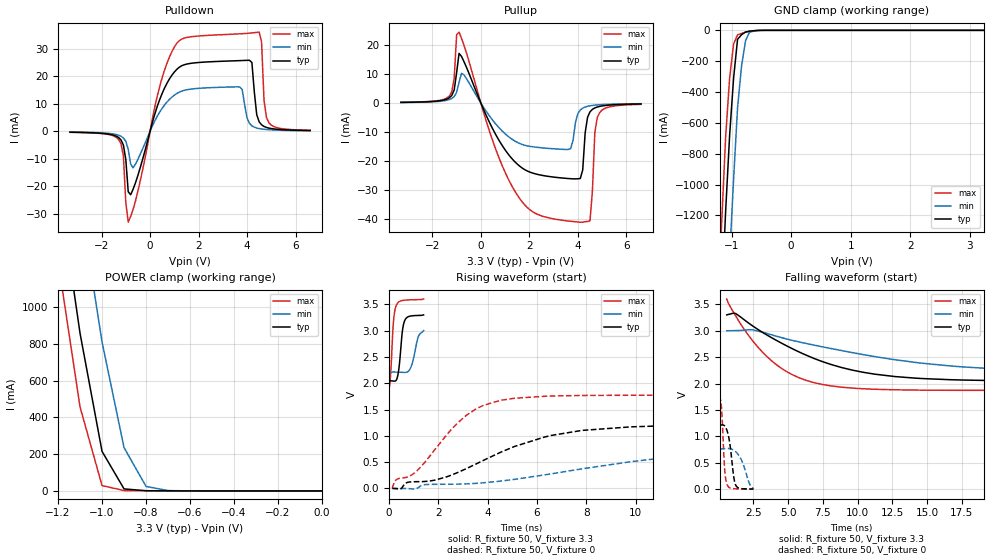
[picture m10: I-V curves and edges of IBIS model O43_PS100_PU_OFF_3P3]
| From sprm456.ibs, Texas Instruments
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|   Model Cell O43_PS100_PU_OFF_3P3
|IDG09_OUO43_PS100_PU_OFF_3P3
[Model]   O43_PS100_PU_OFF_3P3
Model_type   I/O
Polarity   Non-Inverting
Enable   Active-Low
Vinl =  0.8V
Vinh =  2V
Cref =  15pF
Rref =  100.00M
Vref =  0V
Vmeas =  1.65
C_comp   1.7423p   1.5272001p   2.1795998p
[Model Spec]
Vinl   0.8V   0.8V   0.8V
Vinh   2V   2V   2V
[Temperature Range]   25   125   -40
[Voltage Range]   3.3   3   3.6
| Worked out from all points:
|   slope of the pulldown table from 0 to 0.495 V, typ, clamps not added: 36.1 ohm
|   slope of the pullup table from 0 to 0.495 V, typ, clamps not added: 54.7 ohm
|   GND clamp passes 1 mA (typ) near -0.57 V on its own axis
|   POWER clamp passes 1 mA (typ) near -0.79 V on its own axis
|   rising waveform, R_fixture 50, V_fixture 3.3: 20-80 % time 155ps typ, 223ps min, 126ps max; typ from 2.05 V to 3.3 V
|   rising waveform, R_fixture 50, V_fixture 0: 20-80 % time 3.76ns typ, 7.39ns min, 2.05ns max; typ from 0 V to 1.21 V
|   falling waveform, R_fixture 50, V_fixture 3.3: 20-80 % time 6.26ns typ, 10.3ns min, 3.67ns max; typ from 3.3 V to 2.05 V
|   falling waveform, R_fixture 50, V_fixture 0: 20-80 % time 342ps typ, 624ps min, 205ps max; typ from 1.21 V to 0 V
[POWER_clamp]
|   voltage   I(typ)   I(min)   I(max)
-3.3V     22.02A     22.67A     21.68A
-1.2V     1.685A     2.433A     1.254A
-1.167V   1.409A     2.149A     988.2mA
-1.133V   1.134A     1.865A     722.7mA
-1.1V     858.4mA    1.581A     457.2mA
-1.033V   429.7mA    1.068A     171.8mA
-1V       215.3mA    810.7mA    29.13mA
-900mV    11.01mA    235.7mA    2.078mA
-800mV    1.044mA    24.39mA    1.114mA
-700mV    433.7uA    1.869mA    539.5uA
0V        34.07pA    4.936nA    417.4fA
[Pulldown]
|   voltage   I(typ)   I(min)   I(max)
-3.3V     -317uA     -253.1uA   -342.7uA
-1.3V     -2.213mA   -1.382mA   -2.895mA
-1.1V     -4.938mA   -2.395mA   -8.796mA
-900mV    -21.96mA   -6.503mA   -33.05mA
-700mV    -21.08mA   -13.26mA   -28.39mA
1.1V      22.53mA    13.75mA    32mA
3.7V      25.73mA    16.16mA    35.48mA
4.1V      25.87mA    2.915mA    35.73mA
4.5V      3.469mA    1.015mA    36.11mA
4.7V      1.79mA     755.5uA    11.4mA
4.9V      1.19mA     600.1uA    3.153mA
6.6V      301uA      215.6uA    389.3uA
[Pullup]
|   voltage   I(typ)   I(min)   I(max)
-3.3V     241.9uA    204.6uA    268.8uA
-1.3V     1.834mA    1.218mA    2.447mA
-900mV    17.22mA    7.132mA    24.6mA
500mV     -9.137mA   -6.075mA   -13.34mA
1.5V      -21.13mA   -13.59mA   -31.84mA
3.7V      -26.2mA    -15.82mA   -40.94mA
4.1V      -26.12mA   -2.383mA   -41.26mA
4.5V      -3.039mA   -932.7uA   -40.81mA
4.6V      -2.168mA   -805.3uA   -30.41mA
4.7V      -1.674mA   -708uA     -10.08mA
4.9V      -1.143mA   -569.3uA   -3.269mA
6.6V      -301.8uA   -211.1uA   -437.5uA
[GND_clamp]
|   voltage   I(typ)   I(min)   I(max)
-3.3V     -22.41A    -23.18A    -21.98A
-1.233V   -2.33A     -3.195A    -1.825A
-1.167V   -1.743A    -2.601A    -1.246A
-1.1V     -1.172A    -2.017A    -690.4mA
-1.033V   -681.5mA   -1.471A    -309mA
-966.7mV  -310.3mA   -965.9mA   -88.67mA
-900mV    -58.31mA   -501.8mA   -29.31mA
-833.3mV  -28.71mA   -231.8mA   -20.16mA
-766.7mV  -11.17mA   -68.48mA   -12.32mA
-700mV    -5.69mA    -11.83mA   -5.779mA
-433.3mV  -59.55uA   -212.4uA   -19.39uA
3.233V    32.6pA     519.6nA    344.9fA
[Ramp]
| variable   typ   min   max
dV/dt_f 0.77088958/6.3082052n 0.48514794/10.390944n  1.0635239/3.6891142n
dV/dt_r 0.73166814/3.7722821n 0.46348776/7.1613566n  1.0721423/2.0582454n
R_load = 50
[Rising Waveform]
R_fixture = 50
V_fixture = 3.3
V_fixture_min = 3
V_fixture_max = 3.6
|   time   V(typ)   V(min)   V(max)
0s        2.046V     2.211V     1.871V
72.89ps   2.046V     2.212V     2.175V
186.9ps   2.042V     2.212V     3.17V
295.1ps   2.056V     2.211V     3.472V
394.5ps   2.238V     2.21V      3.543V
543.6ps   2.973V     2.208V     3.572V
640.4ps   3.189V     2.206V     3.579V
886.4ps   3.278V     2.298V     3.585V
1.182ns   3.289V     2.871V     3.59V
1.408ns   3.3V       3V         3.6V
[Rising Waveform]
R_fixture = 50
V_fixture = 0
V_fixture_min = 0
V_fixture_max = 0
|   time   V(typ)   V(min)   V(max)
143.3ps   59.65pV    15.83nV    1.384pV
304.9ps   -2.858mV   144.7uV    167.2mV
1.142ns   129.5mV    3.382mV    338.6mV
1.857ns   158.2mV    79.49mV    735.7mV
3.123ns   374.2mV    87.25mV    1.386V
4.514ns   686mV      139.7mV    1.675V
6.303ns   977.9mV    258mV      1.753V
7.807ns   1.103V     372.5mV    1.768V
10.82ns   1.187V     565.1mV    1.773V
18.8ns    1.207V     762.2mV    1.773V
[Falling Waveform]
R_fixture = 50
V_fixture = 3.3
V_fixture_min = 3
V_fixture_max = 3.6
|   time   V(typ)   V(min)   V(max)
581.5ps   3.3V       3V         3.6V
1.232ns   3.325V     3.003V     3.279V
2.287ns   3.121V     3.019V     2.863V
3.494ns   2.916V     2.947V     2.506V
4.879ns   2.716V     2.845V     2.228V
6.644ns   2.499V     2.74V      2.033V
9.629ns   2.254V     2.585V     1.914V
12.69ns   2.132V     2.451V     1.882V
17.65ns   2.066V     2.314V     1.872V
25.58ns   2.046V     2.211V     1.871V
[Falling Waveform]
R_fixture = 50
V_fixture = 0
V_fixture_min = 0
V_fixture_max = 0
|   time   V(typ)   V(min)   V(max)
74.45ps   1.207V     762.2mV    1.773V
225.3ps   1.216V     763mV      1.456V
439ps     1.195V     767.5mV    355.2mV
600.2ps   1.11V      770.2mV    92.75mV
791.9ps   884.3mV    768.2mV    24.49mV
1.081ns   242.7mV    739.7mV    8.528mV
1.217ns   81.95mV    711.8mV    6.619mV
1.66ns    9.282mV    541.5mV    3.277mV
2.201ns   3.771mV    115.3mV    1.578mV
2.495ns   59.65pV    15.83nV    1.384pV
